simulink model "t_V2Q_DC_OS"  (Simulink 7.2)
settings: Solver=ode3  SolverMode=SingleTasking  StartTime=0.0  StopTime=0.005  FixedStep=10e-6  MaxStep=5e-6  RelTol=1e-6  AbsTol=1e-6

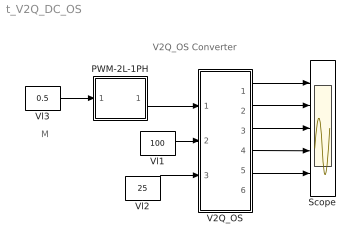
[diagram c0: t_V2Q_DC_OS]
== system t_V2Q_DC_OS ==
  note: V2Q_OS Converter
  note: M
  PWM-2L-1PH : Subsystem  mask(PWM-2L-1PH){FT=2000, PHT=0, DT=1e-6}
      mask prompts: FT "Triangular Frequency"; PHT "Trian. Phase Angle (Degree)"; DT "Dead Time"
      mask help: Pulse Width Modulation for 1 Phase Converter
  Scope : Scope  NumInputPorts=5
  V2Q_OS : Subsystem  mask{L=5e-3, IL0=30, C=1e-4, VC0=50, R=10}
      mask prompts: L "Inductance L"; IL0 "Initial Current"; C "Capacitance C"; VC0 "Initial Cap Voltage VC0"; R "Load Resistance"
      mask help: Voltage two quadrant Converter Input Vector u: u[0]= T1.gate,T2.gate u[1]= E.v u[2]= IDC.i Output Vector y: y[0]= T1.I y[1]= D1.I y[2]= T2.I y[3]= D2.I y[4]= Vo.V y[5]= L1.I y[6]= C1.V y[7]= E.I Parameter Vector p: p[0]= L1.L p[1]= L1.iL0 p[2]= C1.C p[3]= C1.vC0 p[4]= R1.r You can pause the simulation during running, change the Parameters you want and continue the Simulation
  Vl1 : Constant  Value=100
  Vl2 : Constant  Value=25
  Vl3 : Constant  Value=0.5
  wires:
  Vl3/1 -> PWM-2L-1PH/1(In1)
  V2Q_OS/1("iT1, iD1") -> Scope/1
  V2Q_OS/2("iT2, iD2") -> Scope/2
  PWM-2L-1PH/1(Out1) -> V2Q_OS/1(sw)
  Vl1/1 -> V2Q_OS/2(E)
  Vl2/1 -> V2Q_OS/3(EL)
  V2Q_OS/3(vO) -> Scope/3
  V2Q_OS/4(iL) -> Scope/4
  V2Q_OS/5(vC) -> Scope/5

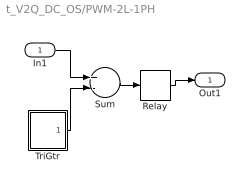
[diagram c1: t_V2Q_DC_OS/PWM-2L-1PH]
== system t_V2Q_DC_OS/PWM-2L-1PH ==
  In1 : Inport  OutDataType=sfix(16)  OutScaling=2^0
  Relay : Relay  OutDataType=sfix(16)  OutScaling=2^0
  Sum : Sum  Inputs=+-  OutDataType=sfix(16)  OutScaling=2^0
  TriGtr : Subsystem  mask(TriGtr){T=1/FT, Td=PHT/FT/360}
      mask prompts: T "Period Time"; Td "Time Delay"
      mask help: Triangular Wave Generator with variable time delay
  Out1 : Outport  InitialOutput=0
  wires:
  In1/1 -> Sum/1
  TriGtr/1(O) -> Sum/2
  Sum/1 -> Relay/1
  Relay/1 -> Out1/1

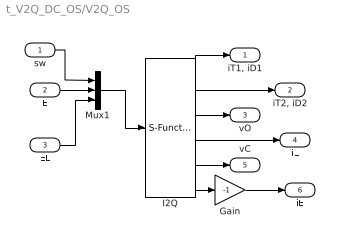
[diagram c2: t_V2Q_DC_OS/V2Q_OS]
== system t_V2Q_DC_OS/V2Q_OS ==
  sw : Inport  OutDataType=sfix(16)  OutScaling=2^0
  E : Inport  Port=2  OutDataType=sfix(16)  OutScaling=2^0
  EL : Inport  Port=3  OutDataType=sfix(16)  OutScaling=2^0
  Gain : Gain  Gain=-1  ParameterDataType=sfix(16)  ParameterScaling=2^0  OutDataType=sfix(16)  OutScaling=2^0
  I2Q : S-Function  FunctionName=s_V2Q_DC_OS  Parameters="[L  IL0 C  VC0  R]"  EnableBusSupport=off
  Mux1 : Mux  Inputs=3
  "iT1, iD1" : Outport  OutDataType=sfix(16)  OutScaling=2^0
  "iT2, iD2" : Outport  Port=2  OutDataType=sfix(16)  OutScaling=2^0
  vO : Outport  Port=3  OutDataType=sfix(16)  OutScaling=2^0
  iL : Outport  Port=4  OutDataType=sfix(16)  OutScaling=2^0
  vC : Outport  Port=5  OutDataType=sfix(16)  OutScaling=2^0
  iE : Outport  Port=6  OutDataType=sfix(16)  OutScaling=2^0
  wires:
  Mux1/1 -> I2Q/1
  sw/1 -> Mux1/1
  E/1 -> Mux1/2
  I2Q/1 -> "iT1, iD1"/1
  I2Q/2 -> "iT2, iD2"/1
  EL/1 -> Mux1/3
  I2Q/5 -> vC/1
  I2Q/6 -> Gain/1
  I2Q/4 -> iL/1
  I2Q/3 -> vO/1
  Gain/1 -> iE/1

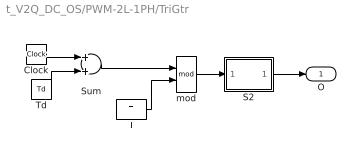
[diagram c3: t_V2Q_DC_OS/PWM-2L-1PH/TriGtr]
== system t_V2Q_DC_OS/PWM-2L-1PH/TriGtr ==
  Clock : Clock
  S2 : Subsystem
  Sum : Sum  OutDataType=sfix(16)  OutScaling=2^0
  T : Constant  Value=T  OutDataType=sfix(16)  OutScaling=2^0
  Td : Constant  Value=Td  OutDataType=sfix(16)  OutScaling=2^0
  mod : Math  Operator=mod
  O : Outport  InitialOutput=0
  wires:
  mod/1 -> S2/1(I1)
  S2/1(O1) -> O/1
  Clock/1 -> Sum/1
  T/1 -> mod/2
  Sum/1 -> mod/1
  Td/1 -> Sum/2

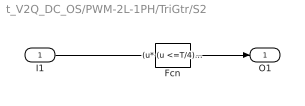
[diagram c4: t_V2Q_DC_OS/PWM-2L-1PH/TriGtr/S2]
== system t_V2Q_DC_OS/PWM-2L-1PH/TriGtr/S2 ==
  I1 : Inport
  Fcn : Fcn  Expr="(u* (u <=T/4) * 4/T)   +  (  (u > T/4) && ( u <=3*T/4) )* ( 1 - (u-T/4) *4/T )   +  ( (u > 3*T/4)&& (u<=T)) * ( ((u -3*T/4)* 4/T )-1 )"
  O1 : Outport
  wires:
  Fcn/1 -> O1/1
  I1/1 -> Fcn/1
